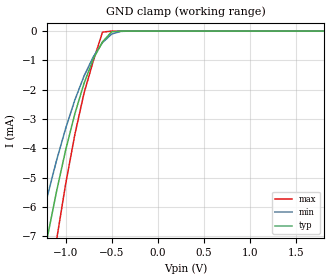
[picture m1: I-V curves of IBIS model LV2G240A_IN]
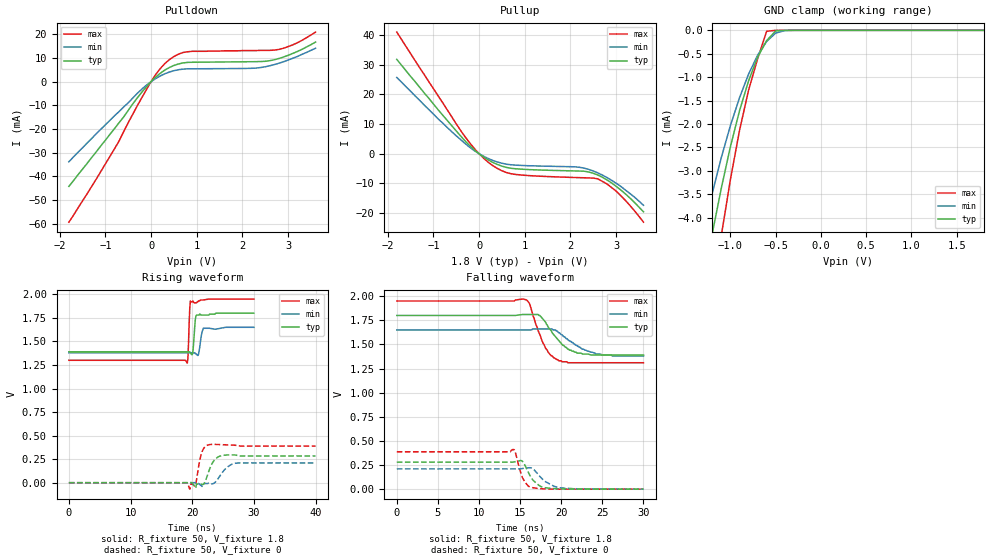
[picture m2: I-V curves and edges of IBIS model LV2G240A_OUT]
|/_/_/_/_/_/_/_/_/_/_/_/_/_/_/_/_/_/_/_/_/_/_/_/_/_/_/_/_/_/_/_/_/_/_/_/_/_/
|   Renesas Electronics Corp.
|   Multi Purpose Semiconductor Digital IC Design Group
|   IBIS Model of HD74LV2G240A
|   1.8V Dual Bus Buffer Inverted with 3-state Outputs,
|   SSOP-8(8pin) Package
|   History
|   V1.0   April   1, 2003   : First release.
|/_/_/_/_/_/_/_/_/_/_/_/_/_/_/_/_/_/_/_/_/_/_/_/_/_/_/_/_/_/_/_/_/_/_/_/_/_/
[IBIS Ver]   2.1
[Comment Char]  |_char
[File name]   l2g240s1.ibs
[File Rev]   1.1
[Date]   April 1, 2003
[Source]   Data created from SPICE simulations at
|   Renesas Electronics Corp.
[Notes]   RLC value of the Package is determined by assuming typical
|   conditions.
[Disclaimer]   This information is for modeling purposes only, and is not
|   guaranteed.
[Copyright]   Copyright 2003, Renesas Electronics Corp.,
|   All Rights Reserved.
|   Component  HD74LV2G240A
[Component]   HD74LV2G240A
[Manufacturer]  Renesas Electronics Corp.
[Package]
|   typ   min   max
R_pkg   0.099   0.095   0.102
L_pkg   1.740nH   1.680nH   1.790nH
C_pkg   0.140pF   0.140pF   0.150pF
[Pin]   signal_name   model_name   R_pin   L_pin   C_pin
1   G1   LV2G240A_IN   0.102   1.780nH   0.140pF
2   A1   LV2G240A_IN   0.097   1.710nH   0.150pF
3   Y2   LV2G240A_OUT   0.095   1.680nH   0.150pF
4   GND   GND   0.102   1.790nH   0.140pF
5   A2   LV2G240A_IN   0.101   1.790nH   0.140pF
6   Y1   LV2G240A_OUT   0.097   1.710nH   0.150pF
7   G2   LV2G240A_IN   0.097   1.710nH   0.150pF
8   VCC   POWER   0.102   1.790nH   0.140pF
| Models and submodels in the file (2): LV2G240A_IN (Input), LV2G240A_OUT (3-state)
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|   Model  LV2G240A_IN
[Model]   LV2G240A_IN
Model_type  Input
Vinl = 0.54V
Vinh = 1.26V
| variable   typ   min   max
C_comp   2.85pF   2.75pF   2.95pF
| variable   typ   min   max
[Temperature range]   25   85   -40
| variable   typ   min   max
[Voltage range]   1.8V   1.65V   1.95V
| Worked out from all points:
|   GND clamp passes 1 mA (typ) near -0.71 V on its own axis
[GND Clamp]
|   Voltage   I(typ)   I(min)   I(max)
-1.8V     -19.4mA    -15.4mA    -25.6mA
-1.3V     -8.81mA    -7.02mA    -11.6mA
-1.2V     -7.07mA    -5.66mA    -9.31mA
-1.1V     -5.49mA    -4.43mA    -7.16mA
-1V       -4.06mA    -3.32mA    -5.22mA
-900mV    -2.82mA    -2.35mA    -3.53mA
-800mV    -1.78mA    -1.53mA    -2.11mA
-700mV    -950uA     -877uA     -1.02mA
-600mV    -366uA     -393uA     -35.6uA
-500mV    -21.6uA    -99uA      -429nA
-400mV    -422nA     -10.2uA    -2.45nA
1.8V      3.69pA     25.5pA     3.6pA
|   Model  LV2G240A_OUT
[Model]   LV2G240A_OUT
Model_type  3-state
Polarity   Inverting
Enable   Active-Low
Vmeas = 0.9V
| variable   typ   min   max
C_comp   7.35pF   7.25pF   7.45pF
| variable   typ   min   max
[Temperature range]   25   85   -40
| variable   typ   min   max
[Voltage range]   1.8V   1.65V   1.95V
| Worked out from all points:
|   slope of the pulldown table from 0 to 0.27 V, typ, clamps not added: 60.6 ohm
|   slope of the pullup table from 0 to 0.27 V, typ, clamps not added: 101 ohm
|   GND clamp passes 1 mA (typ) near -0.78 V on its own axis
|   rising waveform, R_fixture 50, V_fixture 1.8: 20-80 % time 272ps typ, 379ps min, 212ps max; typ from 1.39 V to 1.8 V
|   rising waveform, R_fixture 50, V_fixture 0: 20-80 % time 1.1ns typ, 1.56ns min, 692ps max; typ from 0 V to 0.284 V
|   falling waveform, R_fixture 50, V_fixture 1.8: 20-80 % time 2.32ns typ, 2.98ns min, 1.82ns max; typ from 1.8 V to 1.39 V
|   falling waveform, R_fixture 50, V_fixture 0: 20-80 % time 1.34ns typ, 1.81ns min, 938ps max; typ from 0.28 V to 0 V
[Pullup]
|   Voltage   I(typ)   I(min)   I(max)
-1.8V     31.8mA     25.7mA     41mA
-400mV    5.92mA     4.69mA     7.77mA
-100mV    1.26mA     991uA      1.71mA
200mV     -2.09mA    -1.62mA    -2.86mA
500mV     -4.2mA     -3.22mA    -5.75mA
800mV     -5.08mA    -3.86mA    -7.01mA
2.1V      -5.82mA    -4.43mA    -8.04mA
2.4V      -6.17mA    -5.3mA     -8.18mA
2.6V      -7.2mA     -6.47mA    -8.49mA
3V        -11mA      -9.95mA    -12.6mA
3.3V      -14.9mA    -13.4mA    -17.4mA
3.6V      -19.6mA    -17.4mA    -23.1mA
[Pulldown]
|   Voltage   I(typ)   I(min)   I(max)
-1.8V     -44.2mA    -33.8mA    -59.3mA
-800mV    -19.8mA    -14.4mA    -28.3mA
-200mV    -4.39mA    -3.11mA    -6.66mA
100mV     1.89mA     1.29mA     2.99mA
400mV     5.95mA     4.05mA     9.28mA
600mV     7.46mA     5.03mA     11.6mA
900mV     8.17mA     5.4mA      12.8mA
2.2V      8.4mA      5.62mA     13.1mA
2.6V      8.84mA     6.7mA      13.2mA
2.8V      9.76mA     7.77mA     13.6mA
3.1V      11.9mA     9.85mA     15.5mA
3.6V      16.7mA     14.1mA     20.9mA
[GND Clamp]
|   Voltage   I(typ)   I(min)   I(max)
-1.8V     -11.9mA    -9.46mA    -15.7mA
-1.3V     -5.4mA     -4.31mA    -7.13mA
-1.2V     -4.33mA    -3.47mA    -5.69mA
-1.1V     -3.36mA    -2.71mA    -4.37mA
-1V       -2.48mA    -2.03mA    -3.18mA
-900mV    -1.72mA    -1.44mA    -2.14mA
-800mV    -1.08mA    -936uA     -1.28mA
-700mV    -575uA     -533uA     -610uA
-600mV    -219uA     -237uA     -20.5uA
-500mV    -12.9uA    -58.6uA    -245nA
-400mV    -248nA     -6.13uA    -1.4nA
1.8V      1.91pA     29.2pA     1.8pA
[Ramp]
| variable   typ   min   max
dV/dt_r   0.169/1.081n   0.129/1.625n   0.233/687.4p
dV/dt_f   0.248/2.369n   0.164/2.998n   0.386/1.806n
R_load = 50ohms
[Rising Waveform]
R_fixture = 50
V_fixture = 1.8
V_fixture_min = 1.65
V_fixture_max = 1.95
C_fixture = 0p
|   Time   V(typ)   V(min)   V(max)
0s        1.39V      1.38V      1.3V
19.2ns    1.39V      1.38V      1.27V
19.3ns    1.39V      1.38V      1.32V
19.7ns    1.38V      1.38V      1.93V
20.1ns    1.38V      1.38V      1.93V
20.5ns    1.73V      1.37V      1.91V
20.7ns    1.78V      1.36V      1.91V
21ns      1.78V      1.36V      1.93V
21.8ns    1.78V      1.64V      1.94V
30ns      1.8V       1.65V      1.95V
[Rising Waveform]
R_fixture = 50
V_fixture = 0
C_fixture = 0p
|   Time   V(typ)   V(min)   V(max)
0s        -10.9uV    -28.6uV    -1.96uV
19.1ns    -10.9uV    -28.6uV    -1.96uV
19.6ns    1.13mV     -40.5uV    -68.6mV
20.5ns    -54.1mV    1.3mV      -27.2mV
21.4ns    -13.1mV    -28mV      288mV
22.4ns    66.3mV     -8.99mV    397mV
23.4ns    223mV      -9.61mV    407mV
24.8ns    288mV      101mV      404mV
26.9ns    295mV      206mV      398mV
40ns      284mV      210mV      389mV
[Falling Waveform]
R_fixture = 50
V_fixture = 1.8
V_fixture_min = 1.65
V_fixture_max = 1.95
C_fixture = 0p
|   Time   V(typ)   V(min)   V(max)
0s        1.8V       1.65V      1.95V
15.4ns    1.81V      1.65V      1.97V
16.1ns    1.81V      1.65V      1.93V
17.4ns    1.8V       1.66V      1.6V
18.4ns    1.68V      1.66V      1.42V
19.7ns    1.54V      1.62V      1.33V
21ns      1.44V      1.54V      1.31V
22.6ns    1.4V       1.45V      1.31V
24.2ns    1.39V      1.4V       1.31V
30ns      1.39V      1.38V      1.31V
[Falling Waveform]
R_fixture = 50
V_fixture = 0
C_fixture = 0p
|   Time   V(typ)   V(min)   V(max)
0s        280mV      210mV      387mV
13.8ns    280mV      210mV      387mV
14.2ns    281mV      210mV      412mV
14.4ns    284mV      210mV      385mV
15.3ns    287mV      214mV      117mV
16.2ns    140mV      222mV      21.6mV
17.5ns    28.1mV     123mV      4.92mV
18.1ns    14.2mV     76.3mV     2.18mV
19.8ns    3.16mV     14.3mV     20.2uV
30ns      -21.5uV    -47.8uV    -5.24uV
